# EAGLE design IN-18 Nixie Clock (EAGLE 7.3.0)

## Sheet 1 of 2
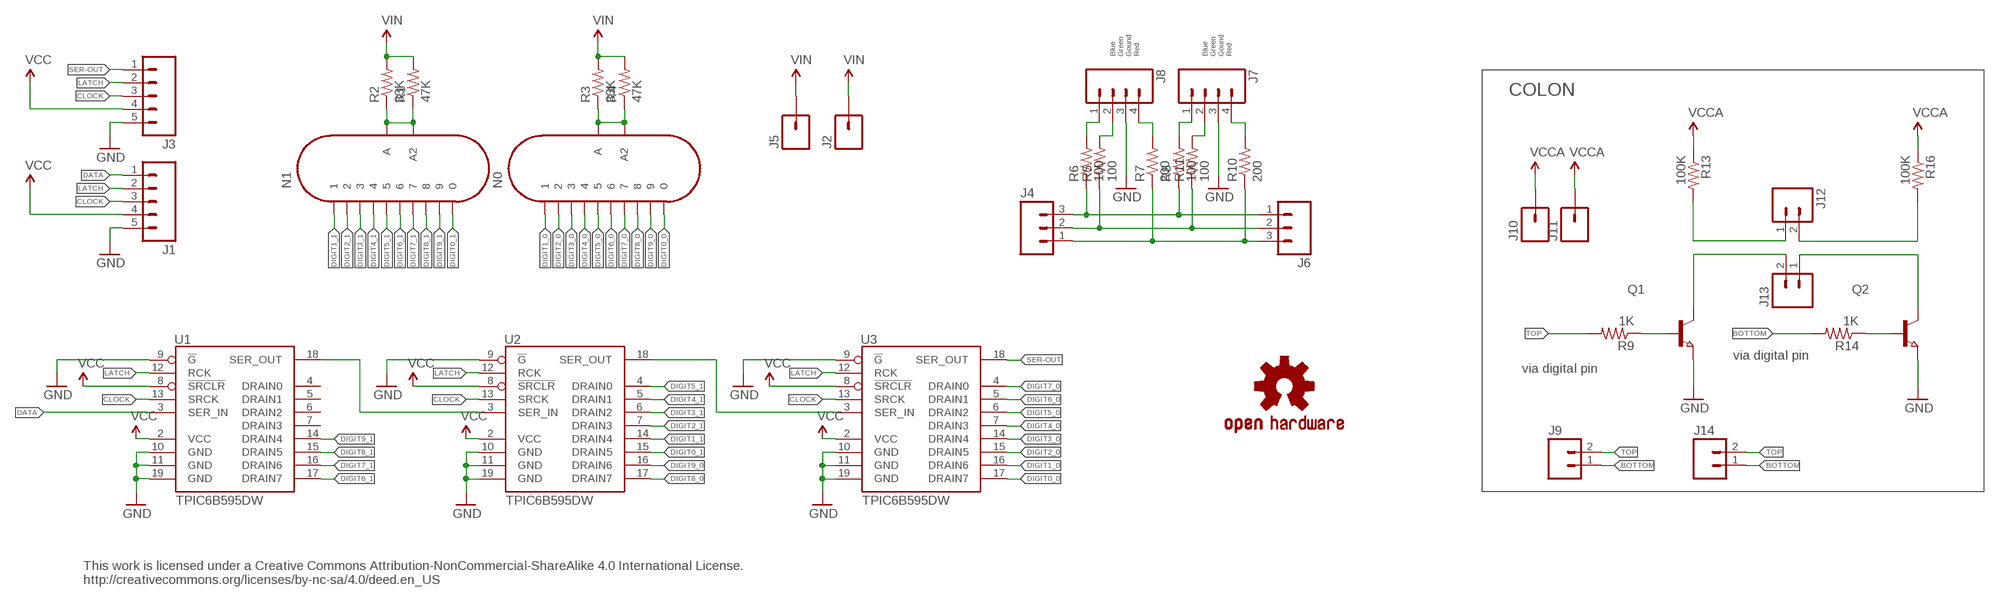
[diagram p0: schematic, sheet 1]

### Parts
J1  M05PTH  [1X05]
J2  M01SMDNS  [1X01NS]
J3  M05PTH  [1X05]
J4  M03PTH  [1X03]
J5  M01SMDNS  [1X01NS]
J6  M03PTH  [1X03]
J7  M04NO_SILK_ALL_ROUND  [1X04_NO_SILK_ALL_ROUND]
J8  M04NO_SILK_ALL_ROUND  [1X04_NO_SILK_ALL_ROUND]
J9  M02PTH  [1X02]
J10  M01SMDNS  [1X01NS]
J11  M01SMDNS  [1X01NS]
J12  M021X02_NO_SILK  [1X02_NO_SILK]
J13  M021X02_NO_SILK  [1X02_NO_SILK]
J14  M02PTH  [1X02]
LOGO1  OSHW-LOGOM  [OSHW-LOGO-M]
N0  IN-18  [IN-18]
N1  IN-18  [IN-18]
Q1  NPN-TRANSISTOR_SOT23  [SOT23]
Q2  NPN-TRANSISTOR_SOT23  [SOT23]
R1  47K  RESISTORPTH-1/2W  [AXIAL-0.5]
R2  33K  RESISTORPTH-1/2W  [AXIAL-0.5]
R3  33K  RESISTORPTH-1/2W  [AXIAL-0.5]
R4  47K  RESISTORPTH-1/2W  [AXIAL-0.5]
R5  100  RESISTOR0805-RES  [0805]
R6  100  RESISTOR0805-RES  [0805]
R7  200  RESISTOR0805-RES  [0805]
R8  100  RESISTOR0805-RES  [0805]
R9  1K  RESISTOR0805-RES  [0805]
R10  200  RESISTOR0805-RES  [0805]
R11  100  RESISTOR0805-RES  [0805]
R13  100K  RESISTORPTH-1/2W  [AXIAL-0.5]
R14  1K  RESISTOR0805-RES  [0805]
R16  100K  RESISTORPTH-1/2W  [AXIAL-0.5]
U1  TPIC6B595DW  [SO20W]
U2  TPIC6B595DW  [SO20W]
U3  TPIC6B595DW  [SO20W]

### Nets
BLUE: J4.3 J6.1 R6.1 R8.1
BOTTOM: J9.1 J14.1 R14.2
CLOCK: J1.3 J3.3 U1.13(SRCK) U2.13(SRCK) U3.13(SRCK)
DATA: J1.1 U1.3(SER_IN)
DIGIT0_0 [hvsup]: N0.0 U3.17(DRAIN7)
DIGIT0_1 [hvsup]: N1.0 U2.15(DRAIN5)
DIGIT1_0 [hvsup]: N0.1 U3.16(DRAIN6)
DIGIT1_1 [hvsup]: N1.1 U2.14(DRAIN4)
DIGIT2_0 [hvsup]: N0.2 U3.15(DRAIN5)
DIGIT2_1: N1.2 U2.7(DRAIN3)
DIGIT3_0 [hvsup]: N0.3 U3.14(DRAIN4)
DIGIT3_1 [hvsup]: N1.3 U2.6(DRAIN2)
DIGIT4_0 [hvsup]: N0.4 U3.7(DRAIN3)
DIGIT4_1 [hvsup]: N1.4 U2.5(DRAIN1)
DIGIT5_0 [hvsup]: N0.5 U3.6(DRAIN2)
DIGIT5_1 [hvsup]: N1.5 U2.4(DRAIN0)
DIGIT6_0 [hvsup]: N0.6 U3.5(DRAIN1)
DIGIT6_1 [hvsup]: N1.6 U1.17(DRAIN7)
DIGIT7_0 [hvsup]: N0.7 U3.4(DRAIN0)
DIGIT7_1 [hvsup]: N1.7 U1.16(DRAIN6)
DIGIT8_0 [hvsup]: N0.8 U2.17(DRAIN7)
DIGIT8_1 [hvsup]: N1.8 U1.15(DRAIN5)
DIGIT9_0 [hvsup]: N0.9 U2.16(DRAIN6)
DIGIT9_1 [hvsup]: N1.9 U1.14(DRAIN4)
GND: J1.5 J3.5 J7.3 J8.3 Q1.2(E) Q2.2(E) U1.9(!G) U1.10(GND) U1.11(GND) U1.19(GND) U2.9(!G) U2.10(GND) U2.11(GND) U2.19(GND) U3.9(!G) U3.10(GND) U3.11(GND) U3.19(GND)
GREEN: J4.2 J6.2 R5.1 R11.1
LATCH: J1.2 J3.2 U1.12(RCK) U2.12(RCK) U3.12(RCK)
N$1: J8.1 R6.2
N$2: N1.A N1.A2 R1.P$1 R2.P$1
N$3: J8.2 R5.2
N$4: J7.2 R11.2
N$5: J7.4 R10.2
N$6: N0.A N0.A2 R3.P$1 R4.P$1
N$7: J8.4 R7.2
N$8: J7.1 R8.2
N$9: Q2.1(B) R14.1
N$11: J13.1 Q2.3(C)
N$12: J12.2 R16.P$2
N$22: Q1.1(B) R9.1
N$23: J12.1 R13.P$2
N$27: U2.18(SER_OUT) U3.3(SER_IN)
N$28: J13.2 Q1.3(C)
N$29: U1.18(SER_OUT) U2.3(SER_IN)
RED: J4.1 J6.3 R7.1 R10.1
SER-OUT: J3.1 U3.18(SER_OUT)
TOP: J9.2 J14.2 R9.2
VCC: J1.4 J3.4 U1.2(VCC) U1.8(!SRCLR) U2.2(VCC) U2.8(!SRCLR) U3.2(VCC) U3.8(!SRCLR)
VCCA: J10.1 J11.1 R13.P$1 R16.P$1
VIN: J2.1 J5.1 R1.P$2 R2.P$2 R3.P$2 R4.P$2
Unconnected: U1.4(DRAIN0) U1.5(DRAIN1) U1.6(DRAIN2) U1.7(DRAIN3)

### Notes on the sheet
- Blue
  Green
  Gound
  Red
- Blue
  Green
  Gound
  Red
- COLON
- via digital pin
- via digital pin
- This work is licensed under a Creative Commons Attribution-NonCommercial-ShareAlike 4.0 International License.
  http://creativecommons.org/licenses/by-nc-sa/4.0/deed.en_US

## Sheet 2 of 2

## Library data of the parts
J1 J3 = SparkFun-Connectors:M05: Header 5 Standard 5-pin 0.1" header. Use with straight break away headers (SKU : PRT-00116), right angle break away headers (PRT-00553), swiss pins (PRT-00743), machine pins (PRT-00117), and female headers (PRT-00115). Molex polarized connector foot print use with SKU : PRT-08230 with associated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
J2 J5 J10 J11 = SparkFun-Connectors:M01: Header 1
J4 J6 = SparkFun-Connectors:M03: Header 3 Standard 3-pin 0.1" header. Use with straight break away headers (SKU : PRT-00116), right angle break away headers (PRT-00553), swiss pins (PRT-00743), machine pins (PRT-00117), and female headers (PRT-00115). Molex polarized connector foot print use with SKU : PRT-08232 with associated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
J7 J8 = SparkFun-Connectors:M04: Header 4 Standard 4-pin 0.1" header. Use with straight break away headers (SKU : PRT-00116), right angle break away headers (PRT-00553), swiss pins (PRT-00743), machine pins (PRT-00117), and female headers (PRT-00115). Molex polarized connector foot print use with SKU : PRT-08231 with associated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; PROD_ID: CONN-09696
J9 J12-J14 = SparkFun-Connectors:M02: Standard 2-pin 0.1" header. Use with
LOGO1 = SparkFun-Aesthetics:OSHW-LOGO: Open Source Hardware Logo
N0 N1 = Nixie Tubes 2:IN-18: IN-18: large numeric frontview nixie tube
Q1 Q2 = semicon-smd-ipc:NPN-TRANSISTOR_: NPN TRANSISTOR
R1-R11 R13 R14 R16 = SparkFun-Resistors:RESISTOR: Resistor
U1-U3 = TPIC6B595:TPIC6B595

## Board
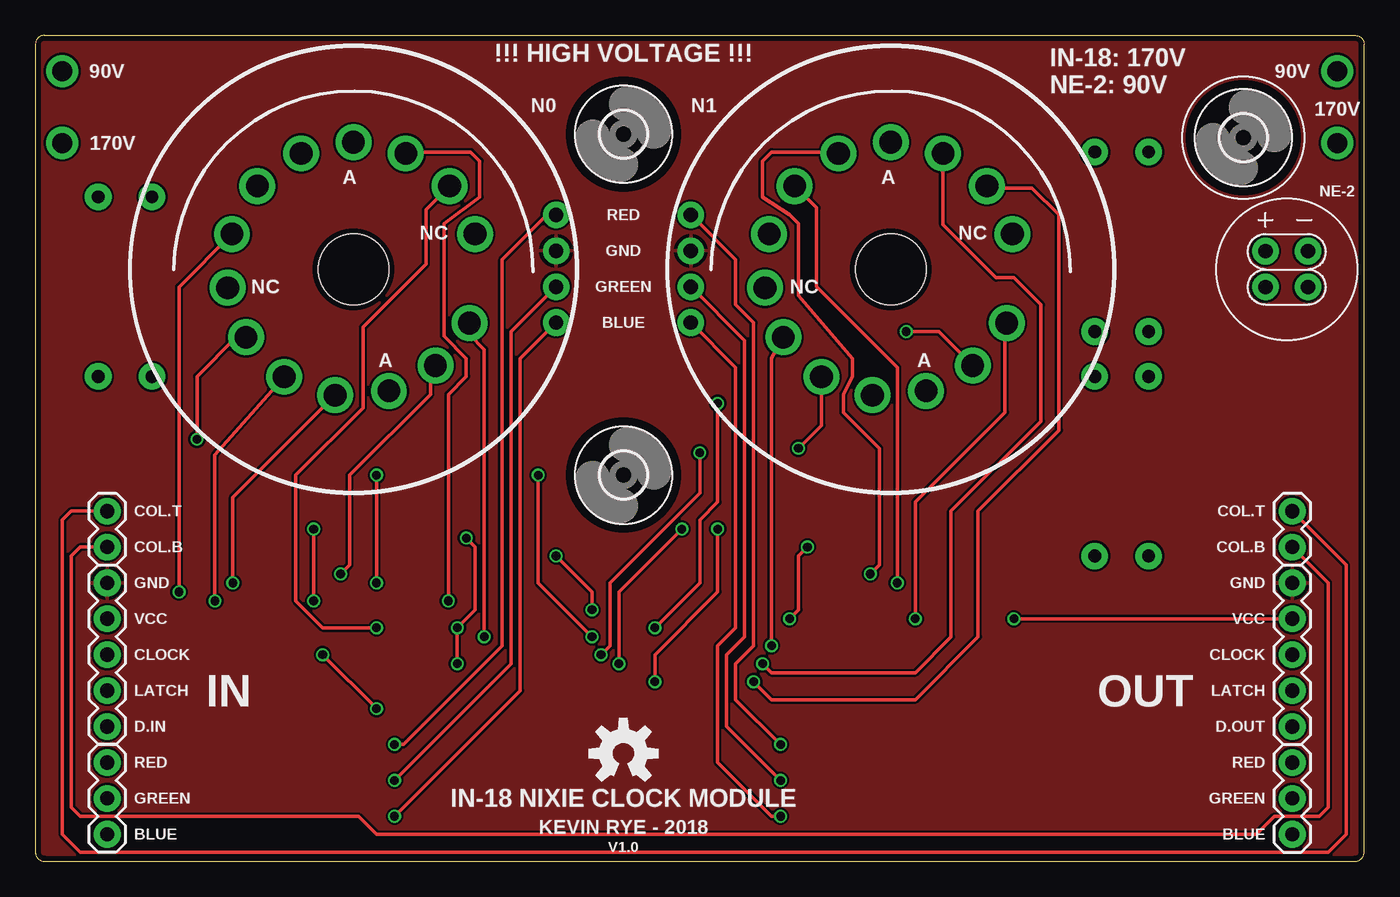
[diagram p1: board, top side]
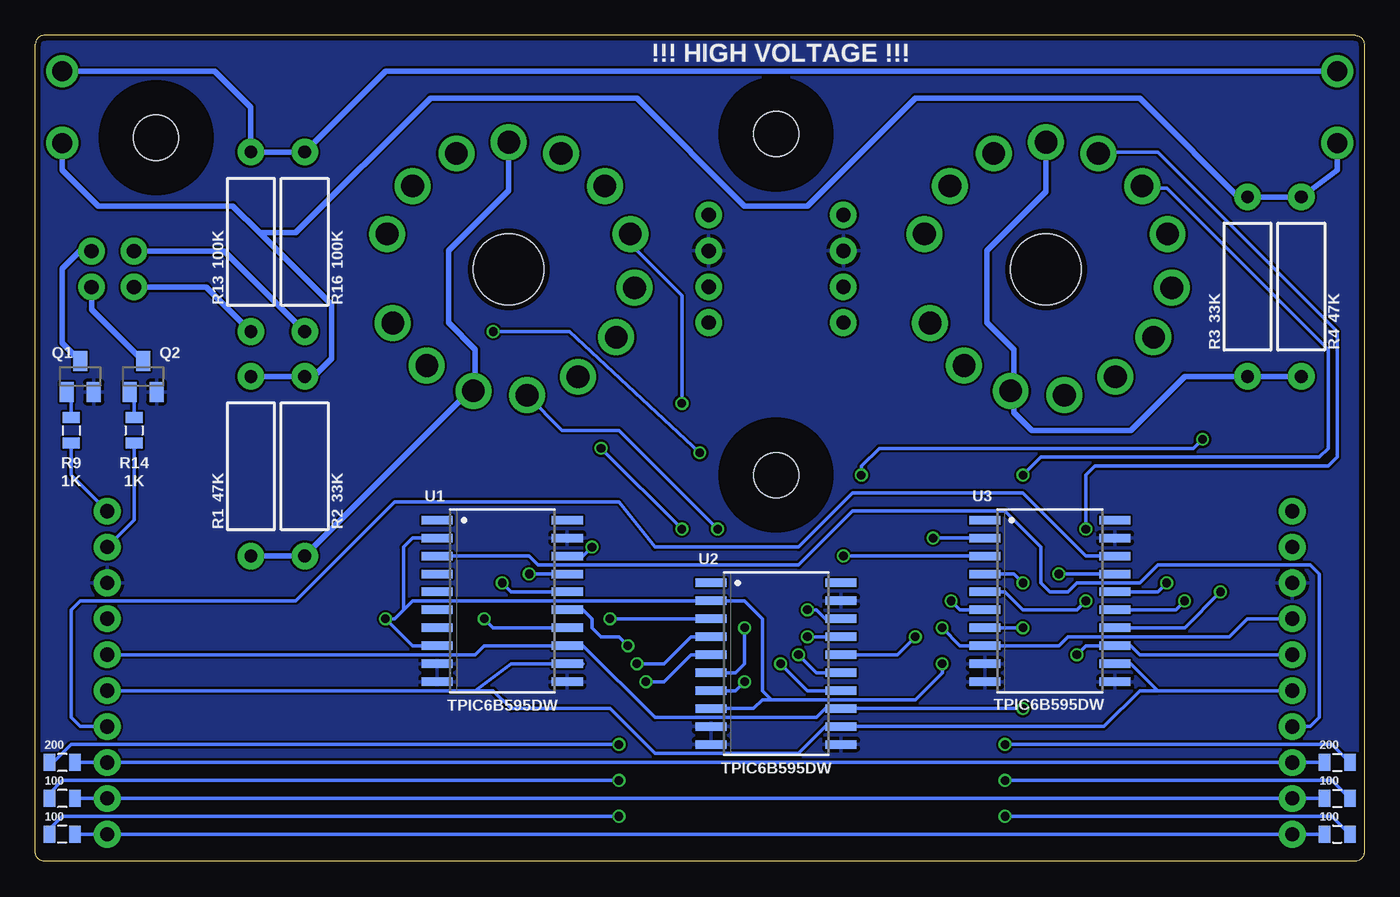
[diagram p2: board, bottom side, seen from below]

Size 93.98 x 58.42 mm. Coordinates in mm from the lower left corner, seen from the top.
Outline: 0.64,58.42 93.34,58.42 arc-90 93.98,57.79 93.98,0.64 arc-90 93.34,0 0.64,0 arc-90 0,0.64 0,57.79 arc-90 0.64,58.42
Copper layers (1*16): Top 0.035559375mm / dielectric 1.6mm / Bottom 0.035559375mm
Design rules "oshpark-2layer": minimum track width 6mil, minimum drill 10mil, track to track 6mil, track to pad 6mil, pad to pad 6mil, via to via 6mil, smd to smd 6mil, copper to edge 15mil, drill to drill 6mil, minimum pad ring 5mil, minimum via ring 5mil, stop-mask expansion 2.5mil, vias tented up to drill 0mil, thermal gap 10mil

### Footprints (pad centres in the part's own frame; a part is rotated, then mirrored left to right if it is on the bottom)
1X05 = drill 1.016 pad 1.88: 1 0,0; 2 2.54,0; 3 5.08,0; 4 7.62,0; 5 10.16,0
1X01NS = drill 1.397 pad 2.286: 1 0,0
1X03 = drill 1.016 pad 1.88: 1 0,0; 2 2.54,0; 3 5.08,0
1X04_NO_SILK_ALL_ROUND = drill 1.016 pad 1.88: 1 0,0; 2 2.54,0; 3 5.08,0; 4 7.62,0
1X02 = drill 1.016 pad 1.88: 1 0,0; 2 2.54,0
1X02_NO_SILK = drill 1.016 pad 1.88: 1 0,0; 2 2.54,0
IN-18 = drill 1.6 pad 2.54: 0 5.8,-6.8; 1 -1.3,-8.9; 2 -4.9,-7.6; 3 -8.6,2.5; 4 6.8,5.9; 5 3.7,8.2; 6 -3.7,8.2; 7 -6.8,5.9; 8 -7.6,-4.8; 9 8.2,-3.8; A 0,9; A2 2.5,-8.6; N/C 8.6,2.5; N/C2 -8.9,-1.3 | hole 5: 0,0
SOT23 = smd 1 x 1.4: 1 -0.95,-1.1; 2 0.95,-1.1; 3 0,1.1
AXIAL-0.5 = drill 0.9 pad 1.88: P$1 -6.35,0; P$2 6.35,0
0805 = smd 0.8 x 1.2: 1 -0.9,0; 2 0.9,0
SO20W = smd 0.6 x 2.2: 1 -5.715,-4.6; 2 -4.445,-4.6; 3 -3.175,-4.6; 4 -1.905,-4.6; 5 -0.635,-4.6; 6 0.635,-4.6; 7 1.905,-4.6; 8 3.175,-4.6; 9 4.445,-4.6; 10 5.715,-4.6; 11 5.715,4.6; 12 4.445,4.6; 13 3.175,4.6; 14 1.905,4.6; 15 0.635,4.6; 16 -0.635,4.6; 17 -1.905,4.6; 18 -3.175,4.6; 19 -4.445,4.6; 20 -5.715,4.6
3,2 = hole 3.2: 0,0

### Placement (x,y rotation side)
J1  5.08,9.53 90 top
J2  92.08,50.8 90 top
J3  88.9,9.53 90 top
J4  5.08,6.99 270 top
J5  1.91,50.8 270 top
J6  88.9,1.91 90 top
J7  36.83,38.1 90 top
J8  46.35,38.1 90 top
J9  88.9,22.22 90 top
J10  92.08,55.88 90 top
J11  1.91,55.88 270 top
J12  87,40.62 90 top
J13  90,40.62 90 top
J14  5.08,22.22 90 top
LOGO1  41.59,7.62 0 top
N0  22.5,41.87 0 top
N1  60.5,41.87 0 top
Q1  90.81,34.29 0 bottom
Q2  86.36,34.29 0 bottom
R1  78.74,27.94 90 bottom
R2  74.93,27.94 90 bottom
R3  8.26,40.64 90 bottom
R4  4.45,40.64 90 bottom
R5  92.08,4.45 180 bottom
R6  92.08,1.91 180 bottom
R7  92.08,6.99 180 bottom
R8  1.91,1.91 0 bottom
R9  91.44,30.48 270 bottom
R10  1.91,6.99 0 bottom
R11  1.91,4.45 0 bottom
R13  78.74,43.82 270 bottom
R14  87,30.48 270 bottom
R16  74.93,43.82 270 bottom
U1  60.96,18.41 270 bottom
U2  41.59,13.97 270 bottom
U3  22.23,18.41 270 bottom
U$2  [3,2]  41.59,27.3 0 top
U$4  [3,2]  41.59,51.44 0 top
U$6  [3,2]  85.44,51.18 0 top

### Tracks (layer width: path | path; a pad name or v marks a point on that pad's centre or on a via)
BLUE
  Bottom 0.254: R8.1 J4.3 J6.1 R6.1
BOTTOM
  Top 0.254: J14.1 3.17,22.22 2.54,21.59 2.54,3.81 3.17,3.17 22.86,3.17 24.13,1.91 86.36,1.91 87.63,3.17 90.81,3.17 91.44,3.81 91.44,19.68 J9.1
  Bottom 0.254: R14.2 87,24.13 J9.1
CLOCK  (via drill 0.61)
  Top 0.254: v20.32,14.61 v24.13,10.79
  Bottom 0.254: J1.3 15.88,14.61 16.51,15.24 U3.13 19.68,15.24 v20.32,14.61 | J3.3 62.87,14.61 62.23,15.24 U1.13 55.24,15.24 50.16,10.16 38.73,10.16 38.1,10.79 U2.13 v24.13,10.79
DATA
  Bottom 0.254: J1.1 3.81,9.53 3.17,10.16 3.17,20.32 3.81,20.95 14.61,20.95 15.88,19.68 20.32,19.68 20.95,19.05 22.23,19.05 22.86,19.68 22.86,22.22 25.4,24.76 36.2,24.76 40.01,20.95 58.42,20.95 59.05,21.59 U1.3
DIGIT0_0  (via drill 0.61)
  Top 0.254: v21.59,20.32 22.23,20.95 22.23,27.3 27.94,33.02 27.94,34.71 N0.0
  Bottom 0.254: U3.17 v21.59,20.32
DIGIT0_1  (via drill 0.61)
  Top 0.254: v40.01,14.61 40.64,15.24 40.64,19.68 46.99,26.04 v46.99,28.89 | v61.59,37.47 63.9,37.47 N1.0
  Bottom 0.254: U2.15 38.73,13.34 v40.01,14.61 | v61.59,37.47 56.2,37.47 v46.99,28.89
DIGIT1_0  (via drill 0.61)
  Top 0.254: v13.97,19.68 13.97,25.73 N0.1
  Bottom 0.254: U3.16 14.61,19.05 v13.97,19.68
DIGIT1_1  (via drill 0.61)
  Top 0.254: v41.27,13.97 41.27,19.05 v45.72,23.49
  Bottom 0.254: U2.14 39.37,12.06 v41.27,13.97 | v45.72,23.49 52.7,30.48 56.72,30.48 N1.1
DIGIT2_0  (via drill 0.61)
  Top 0.254: v12.7,18.41 12.7,28.73 N0.2
  Bottom 0.254: U3.15 13.34,17.78 v12.7,18.41
DIGIT2_1  (via drill 0.61)
  Top 0.254: v43.81,12.7 43.81,14.61 48.26,19.05 v48.26,23.49 | v53.98,29.21 55.6,30.83 N1.2
  Bottom 0.254: U2.7 44.45,12.06 v43.81,12.7 | v48.26,23.49 v53.98,29.21
DIGIT3_0  (via drill 0.61)
  Top 0.254: v10.16,19.05 10.16,40.62 N0.3
  Bottom 0.254: U3.14 12.7,16.51 v10.16,19.05
DIGIT3_1  (via drill 0.61)
  Top 0.254: v43.81,16.51 46.99,19.68 46.99,24.13 48.26,25.4 v48.26,32.39
  Bottom 0.254: U2.6 44.45,13.34 43.81,13.97 v43.81,16.51 | v48.26,32.39 48.26,40.01 51.9,43.65 N1.3
DIGIT4_0  (via drill 0.61)
  Top 0.254: N0.4 27.62,46.09 27.62,42.23 23.18,37.78 23.18,32.07 18.41,27.3 18.41,18.41 20.32,16.51 v24.13,16.51
  Bottom 0.254: v24.13,16.51 U3.7
DIGIT4_1  (via drill 0.61)
  Top 0.254: v50.8,12.7 52.07,11.43 62.23,11.43 66.67,15.88 66.67,24.76 72.39,30.48 72.39,45.72 70.48,47.62 67.44,47.62 N1.4
  Bottom 0.254: U2.5 47.62,14.61 49.53,12.7 v50.8,12.7
DIGIT5_0  (via drill 0.61)
  Top 0.254: v29.21,18.41 29.21,33.02 30.48,34.29 30.48,35.56 28.89,37.15 28.89,45.09 31.43,46.99 31.43,49.53 30.8,50.16 26.3,50.16 N0.5
  Bottom 0.254: U3.6 28.57,17.78 v29.21,18.41
DIGIT5_1  (via drill 0.61)
  Top 0.254: v51.44,13.97 52.07,13.34 62.23,13.34 64.77,15.88 64.77,24.76 71.12,31.11 71.12,39.37 69.22,41.27 67.94,41.27 64.2,45.02 N1.5
  Bottom 0.254: U2.4 47.62,15.88 49.53,13.97 v51.44,13.97
DIGIT6_0  (via drill 0.61)
  Top 0.254: v19.68,18.41 v19.68,23.49
  Bottom 0.254: U3.5 25.4,19.05 24.13,17.78 20.32,17.78 v19.68,18.41 | v19.68,23.49 19.68,27.3 19.05,27.94 2.54,27.94 1.91,28.57 1.91,37.47 14.61,50.16 18.7,50.16 N0.6
DIGIT6_1  (via drill 0.61)
  Top 0.254: v59.05,20.32 59.69,20.95 59.69,29.21 57.15,31.75 57.15,33.02 57.78,34.29 57.78,35.56 53.98,40.01 53.98,45.09 53.34,45.72 51.44,46.99 51.44,49.53 52.07,50.16 56.7,50.16 arc-90 N1.6
  Bottom 0.254: U1.17 v59.05,20.32
DIGIT7_0  (via drill 0.61)
  Top 0.254: v24.13,19.68 v24.13,27.3
  Bottom 0.254: U3.4 24.77,20.32 v24.13,19.68 | v24.13,27.3 22.86,28.57 3.17,28.57 2.54,29.21 2.54,36.2 13.97,47.62 15.56,47.62 N0.7
DIGIT7_1  (via drill 0.61)
  Top 0.254: v60.96,19.68 60.96,34.93 55.24,40.64 55.24,46.22 N1.7
  Bottom 0.254: U1.16 60.33,19.05 v60.96,19.68
DIGIT8_0  (via drill 0.61)
  Top 0.254: N0.8 14.21,37.07 11.43,34.29 v11.43,29.84 | v35.56,27.3 35.56,19.68 v39.37,15.88
  Bottom 0.254: v11.43,29.84 12.06,29.21 34.29,29.21 35.56,27.94 v35.56,27.3 | v39.37,15.88 U2.17
DIGIT8_1  (via drill 0.61)
  Top 0.254: v52.07,15.24 52.07,35.6 N1.8
  Bottom 0.254: U1.15 55.24,17.78 54.61,17.14 54.61,16.51 53.98,15.88 52.7,15.88 v52.07,15.24
DIGIT9_0  (via drill 0.61)
  Top 0.254: N0.9 30.7,37.25 31.75,36.2 v31.75,15.88
  Bottom 0.254: v31.75,15.88 33.02,14.61 U2.16
DIGIT9_1  (via drill 0.61)
  Top 0.254: v62.23,17.14 62.23,25.4 68.58,31.75 68.58,37.95 N1.9
  Bottom 0.254: U1.14 61.59,16.51 v62.23,17.14
GND
  pour Bottom: -0.64,59.05 94.61,59.05 94.61,-0.64 -0.64,-0.64
  pour Top: -1.27,59.69 95.25,59.69 95.25,-1.27 -1.27,-1.27
GREEN
  Bottom 0.254: R11.1 J4.2 J6.2 R5.1
LATCH
  Bottom 0.254: J1.2 14.61,12.06 | 14.61,12.06 16.51,13.97 U3.12 | 55.24,13.97 U1.12 60.33,13.97 62.87,12.06 | 62.87,12.06 J3.2 | 62.87,12.06 61.59,12.06 60.33,10.79 53.34,10.79 50.16,7.62 40.01,7.62 38.1,9.53 U2.12 18.41,9.53 15.88,12.06 14.61,12.06
N$1  (via drill 0.61)
  Top 0.254: v52.7,3.17 52.07,3.17 48.26,6.99 48.26,15.24 49.53,16.51 49.53,34.93 J8.1
  Bottom 0.254: R6.2 92.97,2.28 92.08,3.17 v52.7,3.17
N$2
  Bottom 0.406: R1.P$1 R2.P$1 63.26,33.27 N1.A2 62.87,33.4 62.87,36.2 64.77,38.1 64.77,43.18 60.5,47.45 N1.A
N$3  (via drill 0.61)
  Top 0.254: v52.7,5.71 48.9,9.53 48.9,14.61 50.16,15.88 50.16,36.83 J8.2
  Bottom 0.254: R5.2 92.97,4.82 92.08,5.71 v52.7,5.71
N$4  (via drill 0.61)
  Top 0.254: v25.4,5.71 33.66,13.97 33.66,37.47 J7.2
  Bottom 0.254: R11.2 2.27,5.71 v25.4,5.71
N$5  (via drill 0.61)
  Top 0.254: v25.4,8.26 26.04,8.26 33.02,15.24 33.02,42.55 36.2,45.72 J7.4
  Bottom 0.254: R10.2 2.27,8.26 v25.4,8.26
N$6
  Bottom 0.406: R4.P$1 R3.P$1 12.7,34.29 16.51,30.48 23.5,30.48 24.77,31.75 24.77,33.03 N0.A2 24.77,33.5 24.77,36.2 26.67,38.1 26.67,43.18 22.5,47.35 N0.A
N$7  (via drill 0.61)
  Top 0.254: v52.7,8.26 49.53,11.43 49.53,13.97 50.8,15.24 50.8,38.1 49.53,39.37 49.53,42.55 J8.4
  Bottom 0.254: R7.2 92.71,6.99 91.44,8.26 v52.7,8.26
N$8  (via drill 0.61)
  Top 0.254: v25.4,3.17 34.29,12.06 34.29,35.56 J7.1
  Bottom 0.254: R8.2 2.27,3.17 v25.4,3.17
N$9
  Bottom 0.254: R14.1 87,32.88 Q2.1
N$11
  Bottom 0.406: J13.1 90,39.03 Q2.3
N$12
  Bottom 0.406: J12.2 80.62,43.16 R16.P$2
N$22
  Bottom 0.254: R9.1 91.44,32.88 Q1.1
N$23
  Bottom 0.406: J12.1 81.89,40.62 R13.P$2
N$27  (via drill 0.61)
  Top 0.254: v36.83,21.59 39.37,19.05 v39.37,17.78
  Bottom 0.254: U3.3 v36.83,21.59 | v39.37,17.78 38.73,17.78 38.1,17.14 U2.18
N$28
  Bottom 0.406: J13.2 90.83,43.16 92.08,41.91 92.08,36.66 Q1.3
N$29  (via drill 0.61)
  Top 0.254: v53.34,17.14 53.98,17.78 53.98,21.59 v54.61,22.22
  Bottom 0.254: U2.3 v53.34,17.14 | v54.61,22.22 55.24,21.59 U1.18
RED
  Bottom 0.254: R10.1 J4.1 J6.3 R7.1
SER-OUT
  Bottom 0.254: J3.1 90.81,9.53 91.44,10.16 91.44,17.78 90.81,18.41 75.56,18.41 68.58,25.4 52.7,25.4 50.16,22.22 40.01,22.22 36.2,26.04 24.13,26.04 19.68,21.59 U3.18
TOP
  Top 0.254: J14.2 2.54,24.76 1.91,24.13 1.91,1.91 3.17,0.64 91.44,0.64 92.71,1.91 92.71,20.95 J9.2
  Bottom 0.254: R9.2 91.44,27.3 J9.2
VCC  (via drill 0.61)
  Top 0.254: J3.4 v69.22,17.14 | v30.48,22.86 31.11,22.22 31.11,17.78 v29.84,16.51 v29.84,13.97
  Bottom 0.254: v29.84,16.51 28.57,15.24 U3.8 21.59,15.24 20.95,15.88 9.53,15.88 8.26,17.14 J1.4 | U3.2 v30.48,22.86 | U2.8 43.18,10.79 42.55,11.43 41.91,11.43 | 41.91,11.43 31.75,11.43 29.84,13.34 v29.84,13.97 | 41.91,11.43 42.55,12.06 42.55,17.14 43.81,18.41 U2.2 67.31,18.41 67.94,17.78 | U1.8 67.31,15.24 v69.22,17.14 68.58,17.14 67.94,17.78 | U1.2 67.31,22.86 67.94,22.22 67.94,17.78
VCCA
  Bottom 0.406: J10.1 81.28,55.88 78.74,53.34 R13.P$1 R16.P$1 69.22,55.88 J11.1
VIN
  Bottom 0.406: R1.P$2 R2.P$2 74.3,34.29 73.03,35.56 73.03,39.37 78.11,44.45 | J5.1 1.91,48.9 R4.P$2 R3.P$2 8.26,46.36 15.88,53.98 31.75,53.98 39.37,46.36 43.81,46.36 51.44,53.98 66.04,53.98 75.56,44.45 78.11,44.45 | J2.1 92.08,48.9 89.53,46.36 80.01,46.36 78.11,44.45

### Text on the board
Unrouted: This work is licensed under a Creative Commons Attribution-NonCommercial-ShareAlike 4.0 International License. / http://creativecommons.org/licenses/by-nc-sa/4.0/deed.en_US
tPlace: IN-18: 170V / NE-2: 90V | COL.T | COL.T | COL.B | COL.B | GND | GND | VCC | VCC | CLOCK | CLOCK | LATCH | LATCH | D.IN | D.OUT | RED | RED | GREEN | GREEN | BLUE | BLUE
tNames: 90V | !!! HIGH VOLTAGE !!! | 90V | 170V | 170V | A | A | NE-2 | RED | NC | NC | GND | NC | GREEN | NC | BLUE | A | A | IN | OUT | IN-18 NIXIE CLOCK MODULE | KEVIN RYE - 2018 | V1.0
bNames: !!! HIGH VOLTAGE !!!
